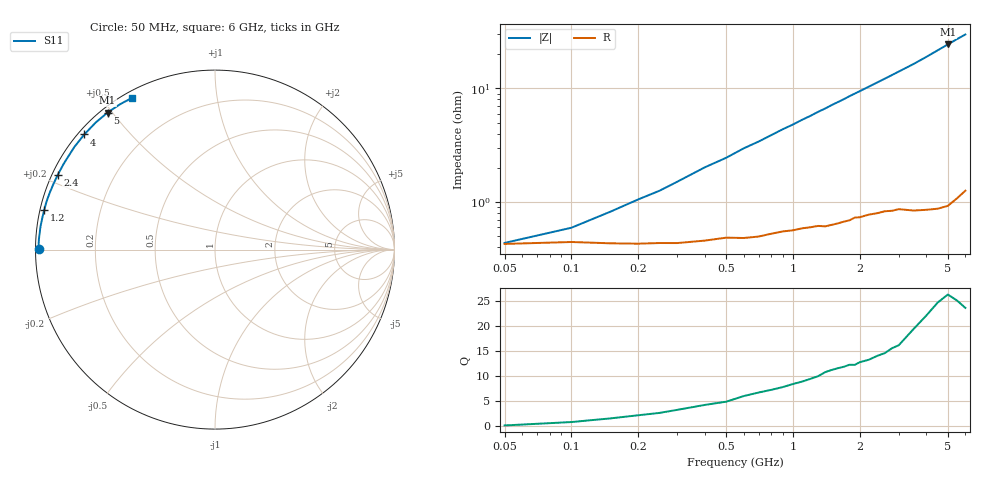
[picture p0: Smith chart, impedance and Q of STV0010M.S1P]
! SIEMENS Discrete & RF Semiconductors
! BA892
! Si PIN Diode in SCD-80
! IF = 10 mA
! S-Parameters:  September  1997
# GHz  S  MA  R  50
!  f  S11
! GHz  MAG  ANG
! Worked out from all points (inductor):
!   34 points, 50 MHz to 6 GHz, reference 50 ohm
!   read as one part to ground: L = 764 pH near 300 MHz
!   highest Q = 25.1 at 5 GHz (marker M1), where L = 774 pH
!   S11 on the Smith chart (normalised r, x): 50 MHz: 0.01, +0.00; 1.2 GHz: 0.01, +0.11; 2.4 GHz: 0.02, +0.22; 4 GHz: 0.02, +0.38; 5 GHz: 0.02, +0.49; 6 GHz: 0.03, +0.59
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0.05  0.983 179.8
0.15  0.9828 178.4
0.2  0.983 177.8
0.25  0.9827 177.3
0.4  0.9819 175.5
0.5  0.9808 174.5
0.6  0.981 173.3
0.7  0.9804 172.3
0.8  0.9793 171.2
0.9  0.9784 170.1
1.1  0.977 168.0
1.2  0.9766 167.0
1.3  0.976 165.9
1.4  0.9763 164.9
1.5  0.9756 163.8
1.6  0.9749 162.8
1.7  0.9741 161.8
1.8  0.9735 160.7
2  0.972 158.7
2.4  0.9701 154.7
2.8  0.9691 150.7
3  0.9684 148.7
3.5  0.9701 143.8
4  0.9706 138.6
4.5  0.971 133.3
5  0.9705 128.1
5.5  0.9672 123.1
6  0.9635 118.5
